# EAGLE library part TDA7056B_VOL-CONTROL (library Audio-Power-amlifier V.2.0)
The TDA7056B is a mono Bridge-Tied Load (BTL) output amplifier with DC volume control. It is designed for use in TV and monitors, but is also suitable for battery-fed portable recorders and radios. The device is contained in a 9-pin medium power package. A Missing Current Limiter (MCL) is built in. The MCL circuit is activated when the difference in current between the output terminal of each amplifier exceeds 100 mA (300 mA typ.). This level of 100 mA allows for headphone applications (single-ended).
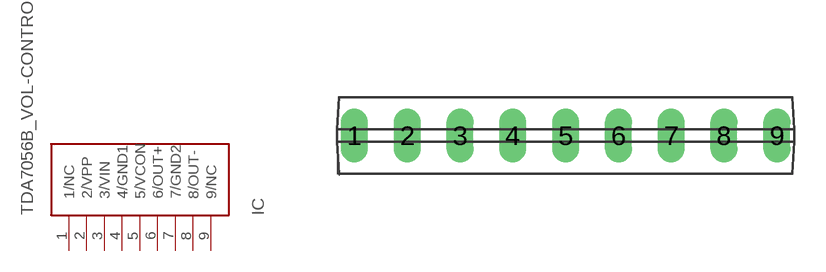
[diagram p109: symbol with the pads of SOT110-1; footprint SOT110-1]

Designator prefix IC

## TDA7056B_VOL-CONTROL  [SOT110-1]
1  1/NC  nc
2  2/VPP  pwr
3  3/VIN  in
4  4/GND1  pwr
5  5/VCON  nc
6  6/OUT+  out
7  7/GND2  pwr
8  8/OUT-  out
9  9/NC  nc

## Footprint SOT110-1 (pad centres in mm)
SIL9MPF: plastic single in-line medium power package with fin; 9 leads
drill 0.8 long: 1 -10.16,0; 2 -7.62,0; 3 -5.08,0; 4 -2.54,0; 5 0,0; 6 2.54,0; 7 5.08,0; 8 7.62,0; 9 10.16,0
